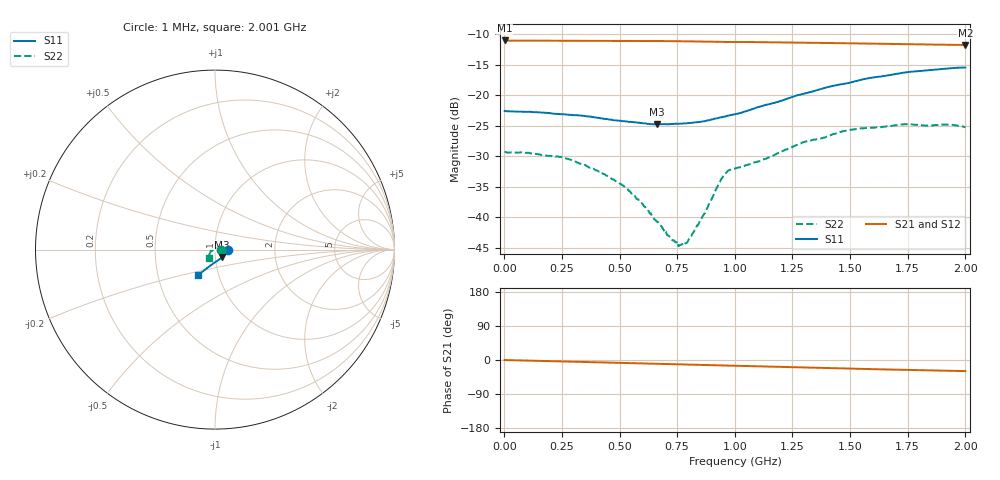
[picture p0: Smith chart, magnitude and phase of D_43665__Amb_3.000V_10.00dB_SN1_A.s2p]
! device id: 43665_
! dir: \\malibu\benchdata\1_engineers\tn_data\43665_75ohm\new\sparar\43665_\amb\3p000v\10p00db
! Serial: 1
! Insertion: A
! Temp: Amb
! VDD: 3.000V
! Attenuation Step: 10.00dB
! IDD: 1.451505e+00mA
! FILE NAME
! DATE 03-27-2009 08:35:48
! CORRECTED  DATA
#  Hz  S  RI  R  75
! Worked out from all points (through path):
!   401 points, 1 MHz to 2.001 GHz, reference 75 ohm
!   highest |S21| = -11.05 dB at 1 MHz (marker M1); lowest = -11.8 dB at 2.001 GHz (marker M2)
!   group delay of S21, straight-line fit = 41.5 ps
!   lowest |S11| = -24.8 dB at 661 MHz (marker M3), VSWR 1.12, Z = 80.8 - j6.82 ohm
!   |S11| at or under -10 dB: start of sweep to end of sweep
!   |S22| runs from -44.7 to -24.7 dB; largest |S21 - S12| = 0.00092
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1000000  0.0743 -0.000655  0.2804 -0.000485  0.2803 -0.000452  0.0344 -0.000297
2.36e8  0.0688 -0.0136  0.279 -0.0172  0.2791 -0.0172  0.03 0.00882
3.36e8  0.0652 -0.0199  0.2781 -0.0245  0.2782 -0.0245  0.0247 0.0115
4.26e8  0.0592 -0.0253  0.2771 -0.031  0.2772 -0.0311  0.0197 0.0116
5.26e8  0.0518 -0.0322  0.2755 -0.0385  0.2756 -0.0386  0.0135 0.0112
6.11e8  0.0443 -0.0383  0.2739 -0.0446  0.2739 -0.0446  0.00669 0.0101
6.61e8  0.0393 -0.0421  0.273 -0.0483  0.273 -0.0483  0.00376 0.00841
6.71e8  0.0387 -0.043  0.2728 -0.0489  0.2728 -0.049  0.00334 0.00818
7.36e8  0.0325 -0.0481  0.2714 -0.0539  0.2714 -0.0538  -0.000847 0.00642
7.66e8  0.0295 -0.0504  0.2706 -0.0561  0.2706 -0.056  -0.00327 0.00496
7.86e8  0.0274 -0.0519  0.2701 -0.0576  0.2701 -0.0576  -0.00492 0.00365
8.21e8  0.0235 -0.0549  0.2691 -0.0603  0.2691 -0.0602  -0.00746 0.0011
8.71e8  0.0173 -0.0587  0.2674 -0.0641  0.2674 -0.0639  -0.0103 -0.00312
9.46e8  0.00831 -0.0656  0.2638 -0.0687  0.264 -0.0685  -0.0194 -0.00802
9.71e8  0.00551 -0.0677  0.2632 -0.0697  0.2634 -0.0696  -0.023 -0.00729
1.001e9  0.00208 -0.0697  0.2628 -0.0713  0.263 -0.0711  -0.0241 -0.007
1.111e9  -0.0125 -0.0797  0.2599 -0.0791  0.2602 -0.0789  -0.0257 -0.0134
1.336e9  -0.0393 -0.0994  0.2517 -0.0933  0.2522 -0.0933  -0.0319 -0.0287
1.491e9  -0.0564 -0.1119  0.2452 -0.1024  0.2455 -0.1025  -0.035 -0.0376
1.671e9  -0.0743 -0.1255  0.2378 -0.1117  0.2379 -0.1121  -0.0351 -0.0431
1.901e9  -0.0904 -0.1368  0.2283 -0.122  0.2281 -0.1221  -0.0348 -0.0457
2.001e9  -0.0944 -0.1392  0.2244 -0.126  0.2238 -0.1267  -0.0323 -0.044
